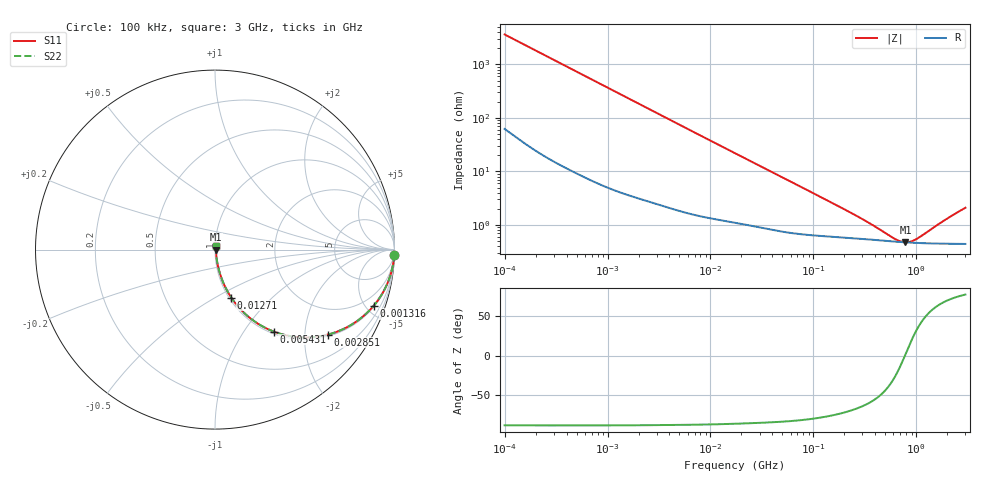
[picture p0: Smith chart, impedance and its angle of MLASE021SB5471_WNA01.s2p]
! MLASE021SB5471_WNA01  S-PARAMETER MODEL  ( Standard Model )
! Model Generated by TAIYO YUDEN Corporation (http://www.ty-top.com)
! Version 1.0
! TAIYO YUDEN Control No. 220901
! Copyright(c) 2022 TAIYO YUDEN CO.,LTD. All Rights Reserved.
! Product Description (link to TY-COMPAS)
! https://ds.yuden.co.jp/TYCOMPAS/or/detail?pn=MLASE021SB5471KWNA01&u=M
! Products Name : Multilayer Ceramic Capacitors
! Characteristics :
!  Capacitance : 470 [pF] , Rated Voltage : 16 [V] , TCC : X5R
!  Case Size : 0.25 x 0.125 / 0.0098 x 0.0049 [mm/inch] , Thickness : 0.125 / 0.0049 [mm/inch]
!  (Conditions: Temperature = 25 [degC] , DC Bias Voltage = 0 [V])
! External Node Assignments :
!  1  o---| |---o  2
! GND o---------o GND
! Frequency Range : 100kHz  -  3GHz  [ 401 STEP ]
# MHZ S RI R 50
! Freq[MHz].  S11 Real  S11 Imag  S21 Real  S21 Imag  S12 Real  S12 Imag  S22 Real  S22 Imag
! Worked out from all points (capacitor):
!   401 points, 100 kHz to 3 GHz, reference 50 ohm
!   read as one part in series: C = 437 pF near 105.3 kHz
!   lowest |Z| = 474 mohm at 785.4 MHz (marker M1)
!   series resonance near 776.6 MHz, so ESL is about 96 pH
!   S11 on the Smith chart (normalised r, x): 100 kHz: 2, -73; 1.316 MHz: 1.08, -5.62; 2.851 MHz: 1.05, -2.61; 5.431 MHz: 1.03, -1.38; 12.71 MHz: 1.02, -0.59; 3 GHz: 1.01, +0.04
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0.1  0.9988 -0.0275  0.00123 0.0275  0.00123 0.0275  0.9988 -0.0275
0.259498  0.9941 -0.0704  0.00589 0.0704  0.00589 0.0704  0.9941 -0.0704
0.562235  0.9754 -0.1488  0.0246 0.1488  0.0246 0.1488  0.9754 -0.1488
0.894104  0.9418 -0.2275  0.0582 0.2275  0.0582 0.2275  0.9418 -0.2275
1.316074  0.884 -0.313  0.116 0.313  0.116 0.313  0.884 -0.313
1.937191  0.7817 -0.4048  0.2183 0.4048  0.2183 0.4048  0.7817 -0.4048
2.851441  0.6276 -0.4738  0.3724 0.4738  0.3724 0.4738  0.6276 -0.4738
3.161081  0.5797 -0.4836  0.4203 0.4836  0.4203 0.4836  0.5797 -0.4836
5.431059  0.3263 -0.4564  0.6737 0.4564  0.6737 0.4564  0.3263 -0.4564
8.202936  0.1812 -0.3698  0.8188 0.3698  0.8188 0.3698  0.1812 -0.3698
12.71297  0.0905 -0.267  0.9095 0.267  0.9095 0.267  0.0905 -0.267
17.7727  0.0531 -0.2002  0.9469 0.2002  0.9469 0.2002  0.0531 -0.2002
37.52708  0.0184 -0.1  0.9816 0.1  0.9816 0.1  0.0184 -0.1
97.38194  0.00793 -0.0392  0.9921 0.0392  0.9921 0.0392  0.00793 -0.0392
287.4592  0.00565 -0.0122  0.9943 0.0122  0.9943 0.0122  0.00565 -0.0122
547.5153  0.00497 -0.00387  0.995 0.00387  0.995 0.00387  0.00497 -0.00387
672.8816  0.00481 -0.00158  0.9952 0.00158  0.9952 0.00158  0.00481 -0.00158
785.4083  0.00472 0.000125  0.9953 -0.000125  0.9953 -0.000125  0.00472 0.000125
893.4279  0.00466 0.00156  0.9953 -0.00156  0.9953 -0.00156  0.00466 0.00156
1016.304  0.00461 0.00303  0.9954 -0.00303  0.9954 -0.00303  0.00461 0.00303
1935.725  0.00459 0.0118  0.9954 -0.0118  0.9954 -0.0118  0.00459 0.0118
3000  0.00483 0.0204  0.9952 -0.0204  0.9952 -0.0204  0.00483 0.0204
